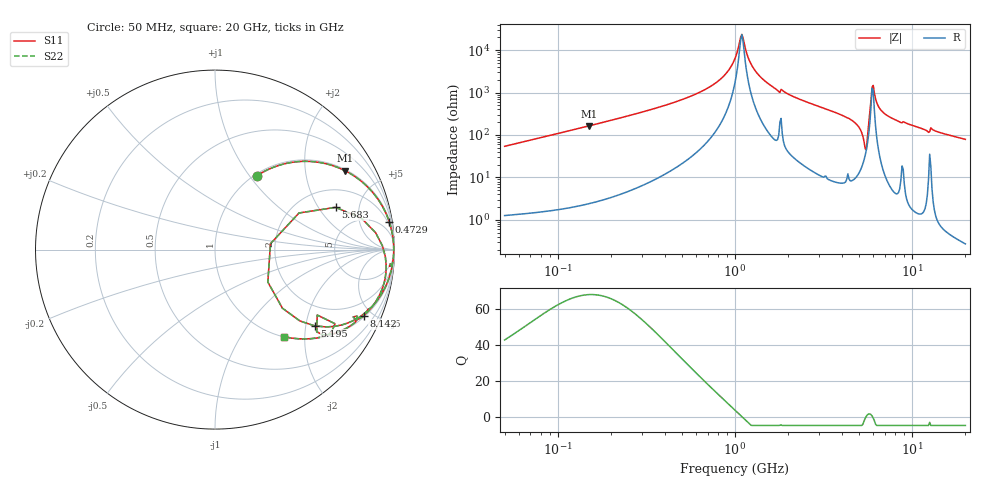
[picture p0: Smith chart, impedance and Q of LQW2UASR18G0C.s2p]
!Murata Part Number: LQW2UASR18G0C
!These Parameters are Measured in Series Mode Connection
!  o--[Z]--o
!Port1  Port2
!  o-------o
!Freq. Start=50[MHz] Stop=20[GHz], 401[Steps]
# Hz S RI R 50
!Freq.(Hz) S11(Real) S11(Imag) S21(Real) S21(Imag) S12(Real) S12(Imag) S22(Real) S22(Imag)
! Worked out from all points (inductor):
!   401 points, 50 MHz to 20 GHz, reference 50 ohm
!   read as one part in series: L = 172 nH near 51.52 MHz
!   highest Q = 68.2 at 149.2 MHz (marker M1), where L = 175 nH
!   self-resonance near 1.078 GHz
!   S11 on the Smith chart (normalised r, x): 50 MHz: 1.03, +1.08; 472.9 MHz: 1, +12; 5.195 GHz: 1.35, -2.25; 5.683 GHz: 3.03, +2.89; 8.142 GHz: 1.08, -4.45; 20 GHz: 1.01, -1.58
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5e7  0.2321 0.4106  0.7679 -0.4106  0.7679 -0.4106  0.2321 0.4106
1.364002e8  0.6874 0.4562  0.3126 -0.4562  0.3126 -0.4562  0.6874 0.4562
1.492265e8  0.7253 0.4391  0.2747 -0.4391  0.2747 -0.4391  0.7253 0.4391
3.721004e8  0.9492 0.2087  0.0508 -0.2087  0.0508 -0.2087  0.9492 0.2087
4.728708e8  0.9708 0.1546  0.0292 -0.1546  0.0292 -0.1546  0.9708 0.1546
7.868965e8  0.9925 0.0564  0.00748 -0.0564  0.00748 -0.0564  0.9925 0.0564
1e9  0.9955 0.015  0.00447 -0.015  0.00447 -0.015  0.9955 0.015
1.094034e9  0.9958 -0.000314  0.00424 0.000314  0.00424 0.000314  0.9958 -0.000314
1.23331e9  0.9953 -0.0208  0.00469 0.0208  0.00469 0.0208  0.9953 -0.0208
1.432596e9  0.9934 -0.0472  0.00655 0.0472  0.00655 0.0472  0.9934 -0.0472
1.740566e9  0.9861 -0.0871  0.0139 0.0871  0.0139 0.0871  0.9861 -0.0871
2.728004e9  0.9621 -0.1783  0.0379 0.1783  0.0379 0.1783  0.9621 -0.1783
4.472136e9  0.8388 -0.3504  0.1612 0.3504  0.1612 0.3504  0.8388 -0.3504
5.194772e9  0.5558 -0.4249  0.4442 0.4249  0.4442 0.4249  0.5558 -0.4249
5.433528e9  0.2945 -0.1812  0.7055 0.1812  0.7055 0.1812  0.2945 -0.1812
5.683258e9  0.672 0.2353  0.328 -0.2353  0.328 -0.2353  0.672 0.2353
5.856089e9  0.8954 0.0933  0.1046 -0.0933  0.1046 -0.0933  0.8954 0.0933
6.034176e9  0.949 -0.0392  0.051 0.0392  0.051 0.0392  0.949 -0.0392
6.601595e9  0.9295 -0.2239  0.0705 0.2239  0.0705 0.2239  0.9295 -0.2239
7.442007e9  0.8721 -0.3221  0.1279 0.3221  0.1279 0.3221  0.8721 -0.3221
8.141811e9  0.8277 -0.3685  0.1723 0.3685  0.1723 0.3685  0.8277 -0.3685
2e10  0.385 -0.4849  0.615 0.4849  0.615 0.4849  0.385 -0.4849
